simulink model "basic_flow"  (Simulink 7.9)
settings: Solver=ode45  StartTime=0.0  StopTime=1000  RelTol=1e-3
libraries: simulink x2

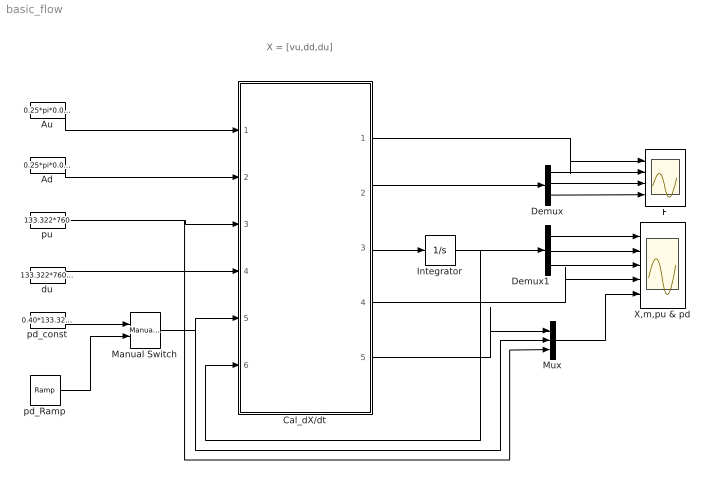
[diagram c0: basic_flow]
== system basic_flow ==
  note: X = [vu,dd,du]
  Ad : Constant  Value=0.25*pi*0.040^2
  Au : Constant  Value=0.25*pi*0.080^2
  Cal_dX/dt : MATLAB Function  TreatAsAtomicUnit=on
  Demux : Demux  Outputs=3
  Demux1 : Demux  Outputs=3
  F : Scope  NumInputPorts=4
  Integrator : Integrator  InitialCondition="[1,  1, 10]"  LimitOutput=on
  Manual Switch : simulink/Signal Routing/Manual Switch  sw=0  action=0  varsize=off
  Mux : Mux  Inputs=3
  X,m,pu & pd : Scope  NumInputPorts=5
  du : Constant  Value=133.322*760/(8.31441/28.96e-3)/(273.15+25.0)
  pd_Ramp : simulink/Sources/Ramp  slope=-133.322*760/1300  start=0  X0=133.322*760
  pd_const : Constant  Value=0.40*133.322*760
  pu : Constant  Value=133.322*760
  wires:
  Cal_dX/dt/3(dX) -> Integrator/1
  Integrator/1 -> Cal_dX/dt/6(X), Demux1/1
  Manual Switch/1 -> Cal_dX/dt/5(pd), Mux/2
  Au/1 -> Cal_dX/dt/1(Au)
  Ad/1 -> Cal_dX/dt/2(Ad)
  pu/1 -> Cal_dX/dt/3(pu), Mux/3
  du/1 -> Cal_dX/dt/4(du)
  Demux1/1 -> X,m,pu & pd/1
  Demux1/2 -> X,m,pu & pd/2
  Demux1/3 -> X,m,pu & pd/3
  Cal_dX/dt/2(F) -> Demux/1
  Demux/1 -> F/2
  Demux/2 -> F/3
  Demux/3 -> F/4
  pd_const/1 -> Manual Switch/1
  pd_Ramp/1 -> Manual Switch/2
  Cal_dX/dt/4(m) -> X,m,pu & pd/4
  Mux/1 -> X,m,pu & pd/5
  Cal_dX/dt/5(pcr) -> Mux/1
  Cal_dX/dt/1(flg) -> F/1

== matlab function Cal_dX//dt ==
function [flg,F,dX,m,pcr] = fcn(Au,Ad,pu,du,pd,X)
A = zeros(3,3);
F = zeros(3,1);
f = 5;

flg = 0;
vu = X(1);
dd = X(2);
vd = X(3);
pcr = pd;

ram1 = diag([1,1,1])*50;
ram2 = diag([1,1,1])*50;
  
F(1) = Au*du*vu-Ad*dd*vd;
F(2) = ((1/2)*(f+2)*pu/du+(1/2)*vu^2)*Au*du*vu-...
    ((1/2)*(f+2)*pd/dd+(1/2)*vd^2)*Ad*dd*vd;
F(3) = Au*pu+Au*du*vu^2-Ad*pd-Ad*dd*vd^2-(Au-Ad)*pu;

A  = zeros(3,3);
A(1, 1) = Au*du;
A(1, 2) = -Ad*vd;
A(1, 3) = -Ad*dd;

A(2, 1) = Au*du*vu^2+((1/2)*(f+2)*pu/du+(1/2)*vu^2)*Au*du;
A(2, 2) = (1/2)*(f+2)*pd*Ad*vd/dd-((1/2)*(f+2)*pd/dd+(1/2)*vd^2)*Ad*vd;
A(2, 3) = -Ad*dd*vd^2-((1/2)*(f+2)*pd/dd+(1/2)*vd^2)*Ad*dd;

A(3, 1) = 2*Au*du*vu;
A(3, 2) = -Ad*vd^2;
A(3, 3) = -2*Ad*dd*vd;

if vd^2 < (f+2)*pd/(f*dd)
    BB = -ram1*F;
    dX = A\BB;
    flg = 1;
else 
    F(1) = Au*du*vu-Ad*dd*vd;
    F(2) = ((1/2)*(f+2)*pu/du+(1/2)*vu^2)*Au*du*vu-((1/2)*f*vd^2+...
        (1/2)*vd^2)*Ad*dd*vd;
    F(3) = Au*pu+Au*du*vu^2-Ad*vd^2*f*dd/(f+2)-Ad*dd*vd^2-(Au-Ad)*pu;
    
    A(1, 1) = Au*du;
    A(1, 2) = -Ad*vd;
    A(1, 3) = -Ad*dd;
    
    A(2, 1) = (1/2)*Au*(3*vu^2*du+pu*f+2*pu);
    A(2, 2) = -(1/2)*vd^3*(f+1)*Ad;
    A(2, 3) = -(3/2)*Ad*dd*vd^2*f-(3/2)*Ad*dd*vd^2;
    
    A(3, 1) = 2*Au*du*vu;
    A(3, 2) = -2*Ad*vd^2*(f+1)/(f+2);
    A(3, 3) = -4*Ad*dd*vd*(f+1)/(f+2);
    pcr = vd^2*f*dd/(f+2);
     
    BB = -ram2*F;
    dX = A\BB;
    flg = -1;
end
m = Ad*dd*vd;
